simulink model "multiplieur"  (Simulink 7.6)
settings: Solver=ode15s  StartTime=0.0  StopTime=0.2  RelTol=1e-3
StopFcn:
  | clc
  | load multiplieur.mat
  | plot(x(1,:),x(2,:),x(1,:),x(3,:),x(1,:),x(4,:))
  | title('entrée, sortie de l''amplificateur et gain d''amplification')
  | axis([0 0.2 -11 11])
  | grid
  | 
  | xlabel('temps')
libraries: fl_lib x5, nesl_utility x4, elec_lib x1

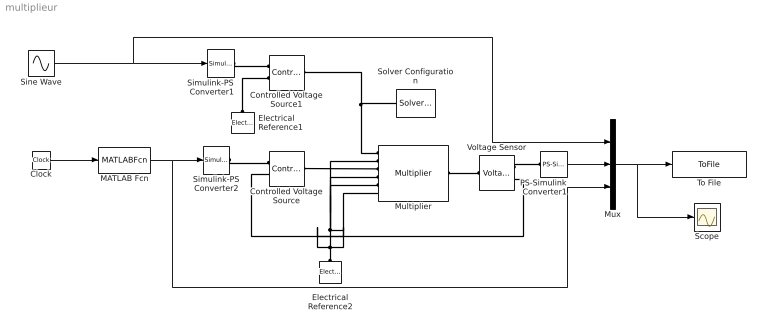
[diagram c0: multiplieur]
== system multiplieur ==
  Clock : Clock
  Controlled Voltage Source : fl_lib/Electrical/Electrical Sources/Controlled Voltage Source  DialogController=NetworkEngine.DynNeDlgSource  SystemSampleTime=-1  i_Log=off  v_Log=off  LocalVarNames=|i|v  LocalVarDescs=|i|v  LocalVarLogging=[0 0]
  Controlled Voltage Source1 : fl_lib/Electrical/Electrical Sources/Controlled Voltage Source  DialogController=NetworkEngine.DynNeDlgSource  SystemSampleTime=-1  i_Log=off  v_Log=off  LocalVarNames=|i|v  LocalVarDescs=|i|v  LocalVarLogging=[0 0]
  Electrical Reference1 : fl_lib/Electrical/Electrical Elements/Electrical Reference  DialogController=NetworkEngine.DynNeDlgSource  SystemSampleTime=-1  i_Log=off  LocalVarNames=|i  LocalVarDescs=|i  LocalVarLogging=[]
  Electrical Reference2 : fl_lib/Electrical/Electrical Elements/Electrical Reference  DialogController=NetworkEngine.DynNeDlgSource  SystemSampleTime=-1  i_Log=off  LocalVarNames=|i  LocalVarDescs=|i  LocalVarLogging=[]
  MATLAB Fcn : MATLABFcn  MATLABFcn=2*(u<=0.05)+5*((0.05<u)&(u<=0.12))+3*(u>0.12)  OutputSignalType=real
  Multiplier : elec_lib/Integrated Circuits/Multiplier  DialogController=NetworkEngine.DynNeDlgSource  SystemSampleTime=-1  K=10 V  A=20  Rin=1e+7 Ohm  Vdiff=10 V  Rout=0.1 Ohm  Vmin=-11 V  Vmax=11 V  Vdotmax=20 V/us  f=1 MHz  V0=0 V  LocalVarLogging=[]
  Mux : Mux  Inputs=3
  PS-Simulink Converter1 : nesl_utility/PS-Simulink Converter  DialogController=NetworkEngine.DynNeUtilDlgSource  SystemSampleTime=-1  PhysicalDomain=network_engine_domain  LeftPortType=input  RightPortType=output  SubClassName=ps_output  Unit=1  AffineConversion=off
  Scope : Scope
  Simulink-PS Converter1 : nesl_utility/Simulink-PS Converter  DialogController=NetworkEngine.DynNeUtilDlgSource  SystemSampleTime=-1  PhysicalDomain=network_engine_domain  LeftPortType=input  RightPortType=output  SubClassName=ps_input  Unit=1  AffineConversion=off  InputFilterTimeConstant=.001  UdotUserProvided=0
  Simulink-PS Converter2 : nesl_utility/Simulink-PS Converter  DialogController=NetworkEngine.DynNeUtilDlgSource  SystemSampleTime=-1  PhysicalDomain=network_engine_domain  LeftPortType=input  RightPortType=output  SubClassName=ps_input  Unit=1  AffineConversion=off  InputFilterTimeConstant=.001  UdotUserProvided=0
  Sine Wave : Sin  Frequency=2*pi*60  SampleTime=0
  Solver Configuration : nesl_utility/Solver Configuration  DialogController=NetworkEngine.DynNeUtilDlgSource  SystemSampleTime=-1  PhysicalDomain=network_engine_domain  LeftPortType=input  RightPortType=generic  SubClassName=solver  Accelerate=off  Profile=off  ResidualTolerance=1e-9  MaxNonlinIter=3  MaxModeIter=2  DoFixedCost=off  UseLocalSampling=off  DoDC=off  LinearAlgebra=Sparse  LocalSolverSampleTime=.001  LocalSolverChoice=NE_BACKWARD_EULER_ADVANCER  UseLocalSolver=off
  To File : ToFile  Filename=multiplieur  MatrixName=x
  Voltage Sensor : fl_lib/Electrical/Electrical Sensors/Voltage Sensor  DialogController=NetworkEngine.DynNeDlgSource  SystemSampleTime=-1  i1_Log=off  v1_Log=off  LocalVarNames=|i1|v1  LocalVarDescs=|i1|v1  LocalVarLogging=[0 0]
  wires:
  Sine Wave/1 -> Simulink-PS Converter1/1, Mux/1
  PS-Simulink Converter1/1 -> Mux/2
  Mux/1 -> To File/1, Scope/1
  Clock/1 -> MATLAB Fcn/1
  MATLAB Fcn/1 -> Simulink-PS Converter2/1, Mux/3
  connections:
  Electrical Reference2/LConn1 -- Multiplier/LConn6 -- Multiplier/LConn5 -- Multiplier/LConn4 -- Multiplier/LConn2 -- Controlled Voltage Source/RConn2 -- Voltage Sensor/RConn2
  Controlled Voltage Source/LConn1 -- Multiplier/LConn3
  Simulink-PS Converter1/RConn1 -- Controlled Voltage Source1/RConn1
  Electrical Reference1/LConn1 -- Controlled Voltage Source1/RConn2
  Simulink-PS Converter2/RConn1 -- Controlled Voltage Source/RConn1
  Multiplier/LConn1 -- Controlled Voltage Source1/LConn1 -- Solver Configuration/RConn1
  Multiplier/RConn1 -- Voltage Sensor/LConn1
  Voltage Sensor/RConn1 -- PS-Simulink Converter1/LConn1
